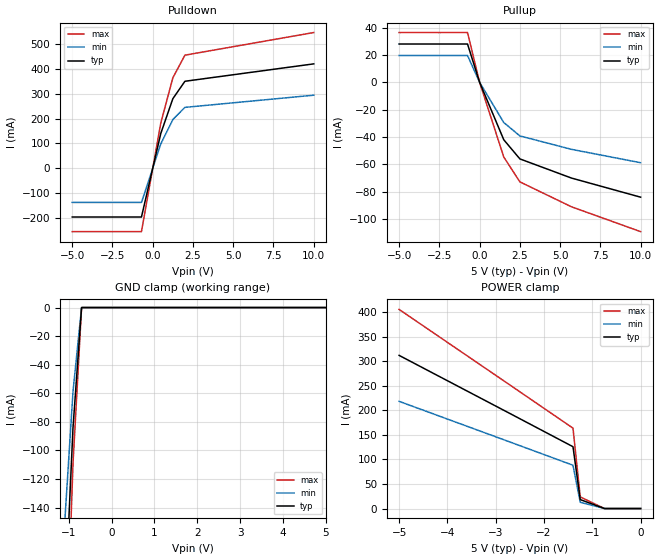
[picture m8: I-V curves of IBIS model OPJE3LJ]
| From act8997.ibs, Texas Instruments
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[Model]   OPJE3LJ
| 48-mA 3-state CMOS/TTL output buffer with 0.5 di/dt and active-low enable
| OP (97318 ALEY)
| BP (97318 ALEY)
Model_type   3-state
Polarity   Non-Inverting
| Signals   DTCK
| variable   typ   min   max
C_comp   10pF   NA   NA
| variable   typ   min   max
[Voltage range]   5.0V   4.5V   5.5V
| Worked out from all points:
|   slope of the pulldown table from 0 to 0.75 V, typ, clamps not added: 4.02 ohm
|   slope of the pullup table from 0 to 0.75 V, typ, clamps not added: 35.7 ohm
|   GND clamp passes 1 mA (typ) near -0.70 V on its own axis
[pullup]
|   50C:5V:   100C:4.5V:weak  0C:5.5V:strong
| Voltage   I(typ)   I(min)   I(max)
-5V       28mA       19.6mA     36.4mA
-2.75V    28mA       19.6mA     36.4mA
-1.4V     28mA       19.6mA     36.4mA
-1.25V    28mA       19.6mA     36.4mA
-750mV    28mA       19.6mA     36.4mA
0V        0A         0A         0A
1.5V      -42mA      -29.4mA    -54.6mA
2.5V      -56mA      -39.2mA    -72.8mA
5.7V      -70mA      -49mA      -91mA
10V       -84mA      -58.8mA    -109.2mA
[pulldown]
|   50C:5V:   100C:4.5V:weak  0C:5.5V:strong
| Voltage   I(typ)   I(min)   I(max)
-5V       -196mA     -137.2mA   -254.8mA
-900mV    -196mA     -137.2mA   -254.8mA
-700mV    -196mA     -137.2mA   -254.8mA
-500mV    -140mA     -98mA      -182mA
0V        0A         0A         0A
500mV     140mA      98mA       182mA
1.25V     280mA      196mA      364mA
2V        350mA      245mA      455mA
10V       420mA      294mA      546mA
[power_clamp]
|   50C:5V:   100C:4.5V:weak  0C:5.5V:strong
| Voltage   I(typ)   I(min)   I(max)
-5V       312.2mA    218.5mA    405.9mA
-2.75V    196mA      137.2mA    254.8mA
-1.4V     126mA      88.2mA     163.8mA
-1.25V    18.2mA     12.7mA     23.7mA
-750mV    0A         0A         0A
0V        0A         0A         0A
[gnd_clamp]
|   50C:5V:   100C:4.5V:weak  0C:5.5V:strong
| Voltage   I(typ)   I(min)   I(max)
-5V       -2.8A      -2A        -3.6A
-900mV    -84mA      -58.8mA    -109.2mA
-700mV    0A         0A         0A
0V        0A         0A         0A
5V        0A         0A         0A
[ramp]
| variable   typ   min   max
dV/dt_r   1.5/1.5e-9   1.2/2.25e-9   1.8/1e-9
dV/dt_f   2.7/2e-9   2.3/3e-9   3.1/1.33e-9
